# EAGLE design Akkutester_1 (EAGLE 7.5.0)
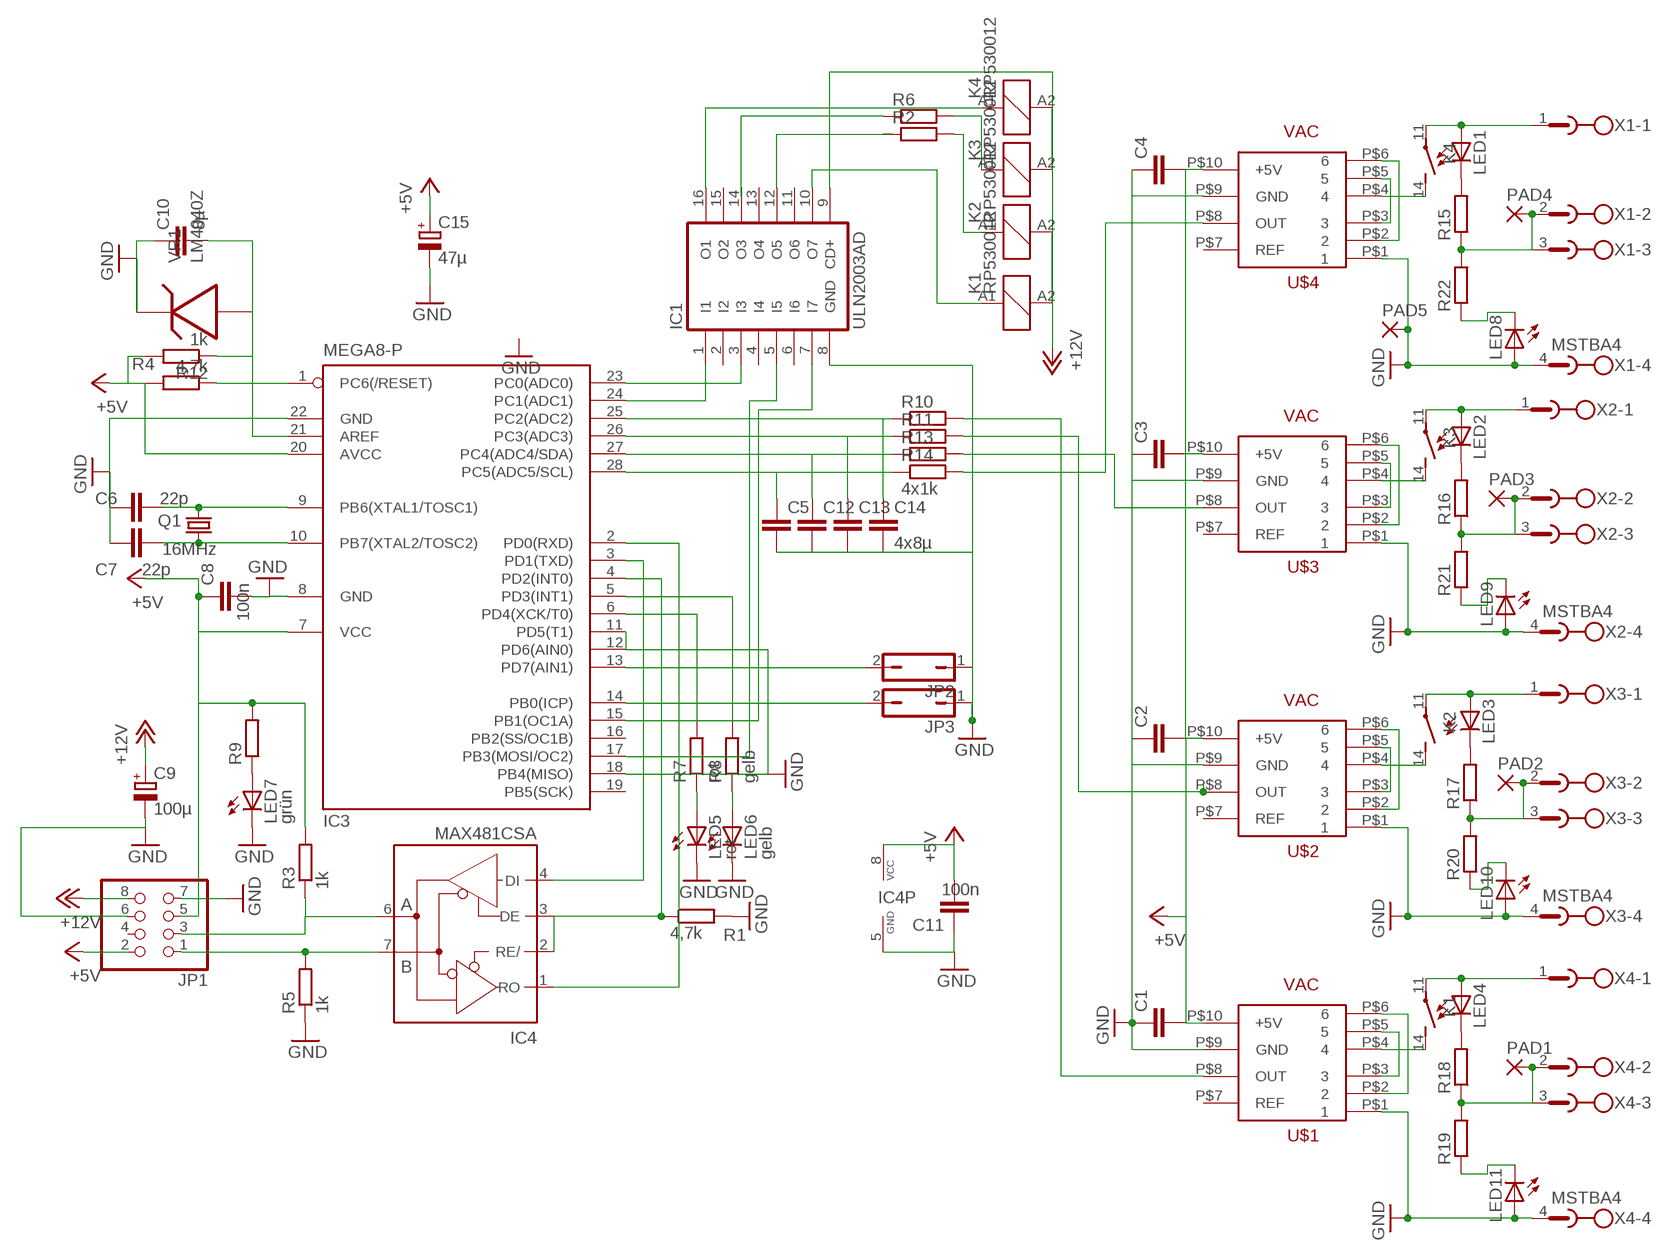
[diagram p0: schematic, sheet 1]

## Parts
C1  C-EUC0805  [C0805]
C2  C-EUC0805  [C0805]
C3  C-EUC0805  [C0805]
C4  C-EUC0805  [C0805]
C5  C-EUC0805  [C0805]
C6  22p  C-EUC0603  [C0603]
C7  22p  C-EUC0603  [C0603]
C8  100n  C-EUC0603  [C0603]
C9  100µ  CPOL-EUSMCD  [SMC_D]
C10  8µ  C-EUC0805  [C0805]
C11  100n  C-EU050-025X075  [C050-025X075]
C12  C-EUC0805  [C0805]
C13  C-EUC0805  [C0805]
C14  4x8µ  C-EUC0805  [C0805]
C15  47µ  CPOL-EUSMCD  [SMC_D]
IC1  ULN2003AD  [SO16]
IC3  MEGA8-P  [DIL28-3]
IC4  MAX481CSA  [SO08]
JP1  PINHD-2X4  [2X04]
JP2  JP1Q  [JP1]
JP3  JP1Q  [JP1]
K1  RP530012  [RP53]
K2  RP530012  [RP53]
K3  RP530012  [RP53]
K4  RP530012  [RP53]
LED1  LED3MM  [LED3MM]
LED2  LED3MM  [LED3MM]
LED3  LED3MM  [LED3MM]
LED4  LED3MM  [LED3MM]
LED5  rot  LEDCHIPLED_0603  [CHIPLED_0603]
LED6  gelb  LEDCHIPLED_0603  [CHIPLED_0603]
LED7  grün  LEDCHIPLED_0603  [CHIPLED_0603]
LED8  LED3MM  [LED3MM]
LED9  LED3MM  [LED3MM]
LED10  LED3MM  [LED3MM]
LED11  LED3MM  [LED3MM]
PAD1  1,6/0,9  [1,6/0,9]
PAD2  1,6/0,9  [1,6/0,9]
PAD3  1,6/0,9  [1,6/0,9]
PAD4  1,6/0,9  [1,6/0,9]
PAD5  1,6/0,9  [1,6/0,9]
Q1  16MHz  CRYSTALCTS406  [CTS406]
R1  4,7k  R-EU_R0603  [R0603]
R2  R-EU_R1206  [R1206]
R3  1k  R-EU_R0603  [R0603]
R4  4,7k  R-EU_R0603  [R0603]
R5  1k  R-EU_R1206  [R1206]
R6  R-EU_R1206  [R1206]
R7  rot  R-EU_R0603  [R0603]
R8  gelb  R-EU_R0603  [R0603]
R9  R-EU_R0603  [R0603]
R10  R-EU_R0603  [R0603]
R11  R-EU_R0603  [R0603]
R12  1k  R-EU_R0603  [R0603]
R13  R-EU_R0603  [R0603]
R14  4x1k  R-EU_R0603  [R0603]
R15  R-EU_R0603  [R0603]
R16  R-EU_R0603  [R0603]
R17  R-EU_R0603  [R0603]
R18  R-EU_R0603  [R0603]
R19  R-EU_R0603  [R0603]
R20  R-EU_R0603  [R0603]
R21  R-EU_R0603  [R0603]
R22  R-EU_R0603  [R0603]
U$1  VAC  [VAC]
U$2  VAC  [VAC]
U$3  VAC  [VAC]
U$4  VAC  [VAC]
VR1  LM4040Z  [TO92]
X1  MSTBA4  [MSTBA4]
X2  MSTBA4  [MSTBA4]
X3  MSTBA4  [MSTBA4]
X4  MSTBA4  [MSTBA4]

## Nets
+5V: C1.2 C2.2 C3.2 C4.2 C8.1 C11.2 C15.+ IC3.7(VCC) IC3.20(AVCC) IC4.8(VCC) JP1.2 JP1.5 R3.2 R4.2 R9.2 R12.2 U$1.P$10(+5V) U$2.P$10(+5V) U$3.P$10(+5V) U$4.P$10(+5V)
+12V: C9.+ IC1.9(CD+) JP1.8 K1.A2 K2.A2 K3.A2 K4.A2
GND: C1.1 C2.1 C3.1 C4.1 C5.2 C6.1 C7.1 C8.2 C9.- C10.1 C11.1 C12.2 C13.2 C14.2 C15.- IC1.8(GND) IC3.8(GND) IC3.11(PD5(T1)) IC3.12(PD6(AIN0)) IC3.18(PB4(MISO)) IC3.22(GND) IC4.5(GND) JP1.6 JP1.7 JP2.1 JP3.1 LED5.C LED6.C LED7.C LED8.A LED9.A LED10.A LED11.A PAD5.1(P) R1.2 R5.1 U$1.P$1 U$1.P$9(GND) U$2.P$1 U$2.P$9(GND) U$3.P$1 U$3.P$9(GND) U$4.P$1 U$4.P$9(GND) VR1.1 X1.4 X2.4 X3.4 X4.4
N$1: R14.2 U$4.P$8(OUT)
N$2: K1.14(2:S) U$1.P$4
N$3: IC1.1(I1) IC3.24(PC1(ADC1))
N$4: R11.2 U$2.P$8(OUT)
N$5: R10.2 U$1.P$8(OUT)
N$6: U$1.P$3 U$1.P$5
N$7: U$1.P$2 U$1.P$6
N$9: K2.14(2:S) U$2.P$4
N$10: U$2.P$3 U$2.P$5
N$11: U$2.P$2 U$2.P$6
N$13: K3.14(2:S) U$3.P$4
N$14: U$3.P$3 U$3.P$5
N$15: U$3.P$2 U$3.P$6
N$17: K4.11(2:P) LED1.A X1.1
N$18: PAD3.1(P) R16.1 R21.2 X2.2 X2.3
N$19: LED2.K(C) R16.2
N$20: K4.14(2:S) U$4.P$4
N$21: R13.2 U$3.P$8(OUT)
N$22: IC1.16(O1) K4.A1
N$23: K3.11(2:P) LED2.A X2.1
N$24: K2.11(2:P) LED3.A X3.1
N$25: K1.11(2:P) LED4.A X4.1
N$26: LED1.K(C) R15.2
N$28: IC4.6(A) JP1.3 R3.1
N$29: IC1.3(I3) IC3.23(PC0(ADC0))
N$30: C7.2 IC3.10(PB7(XTAL2/TOSC2)) Q1.1
N$31: U$4.P$3 U$4.P$5
N$32: U$4.P$2 U$4.P$6
N$33: PAD1.1(P) R18.1 R19.2 X4.2 X4.3
N$34: C6.2 IC3.9(PB6(XTAL1/TOSC1)) Q1.3
N$35: IC3.4(PD2(INT0)) IC4.2(RE/) IC4.3(DE) R1.1
N$36: IC3.1(PC6(/RESET)) R4.1
N$37: IC3.2(PD0(RXD)) IC4.1(RO)
N$38: IC3.3(PD1(TXD)) IC4.4(DI)
N$39: IC3.14(PB0(ICP)) JP3.2
N$40: IC3.13(PD7(AIN1)) JP2.2
N$41: IC3.6(PD4(XCK/T0)) R7.2
N$42: IC3.5(PD3(INT1)) R8.2
N$43: LED5.A R7.1
N$44: LED6.A R8.1
N$45: K2.A1 R2.2
N$46: IC1.5(I5) IC3.17(PB3(MOSI/OC2))
N$47: IC1.7(I7) IC3.15(PB1(OC1A))
N$48: LED7.A R9.1
N$49: IC1.14(O3) R6.1
N$50: IC1.10(O7) K1.A1
N$51: C10.2 IC3.21(AREF) R12.1 VR1.2
N$52: IC1.12(O5) R2.1
N$53: C14.1 IC3.25(PC2(ADC2)) R10.1
N$54: K3.A1 R6.2
N$55: C13.1 IC3.26(PC3(ADC3)) R11.1
N$56: C12.1 IC3.27(PC4(ADC4/SDA)) R13.1
N$57: C5.1 IC3.28(PC5(ADC5/SCL)) R14.1
N$58: IC4.7(B) JP1.1 R5.2
N$59: PAD4.1(P) R15.1 R22.2 X1.2 X1.3
N$60: PAD2.1(P) R17.1 R20.2 X3.2 X3.3
N$61: LED3.K(C) R17.2
N$62: LED4.K(C) R18.2
N$63: LED11.K(C) R19.1
N$64: LED10.K(C) R20.1
N$65: LED9.K(C) R21.1
N$66: LED8.K(C) R22.1
Unconnected: IC1.2(I2) IC1.4(I4) IC1.6(I6) IC1.11(O6) IC1.13(O4) IC1.15(O2) IC3.16(PB2(SS/OC1B)) IC3.19(PB5(SCK)) JP1.4 U$1.P$7(REF) U$2.P$7(REF) U$3.P$7(REF) U$4.P$7(REF)

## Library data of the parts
C1-C8 C10-C14 = rcl:C-EU: CAPACITOR, European symbol
C9 C15 = rcl:CPOL-EU: POLARIZED CAPACITOR, European symbol
IC1 = uln-udn:ULN2003A: DRIVER ARRAY
IC3 = atmel:MEGA8-P: MICROCONTROLLER 8 Kbytes FLASH, 1 kbytes SRAM, 512 bytes EEPROM, USART, 4-channel 10 bit ADC, 2-channel 8 bit ADC Pin compatible with Atmega48, ATMega88, ATMega168 Source: avr.lbr
IC4 = maxim:MAX481CSA: RS485 TRANSEIVER
JP1 = pinhead:PINHD-2X4: PIN HEADER
JP2 JP3 = jumper:JP1Q: JUMPER
K1-K4 = relay:RP53*: Power PCB Relay RP I SCHRACK 1 pole 8 A Vertical version Source: http://www.schrack.com/.. 5845.pdf
LED1-LED11 = led:LED: LED
PAD1-PAD5 = wirepad:1,6/0,9: THROUGH-HOLE PAD
Q1 = crystal:CRYSTAL: CRYSTAL
R1-R22 = rcl:R-EU_: RESISTOR, European symbol
U$1-U$4 = VAC:VAC
VR1 = synthdiy:LM4040: Shunt VOLTAGE REG.
X1-X4 = con-phoenix-508:MSTBA4: PHOENIX

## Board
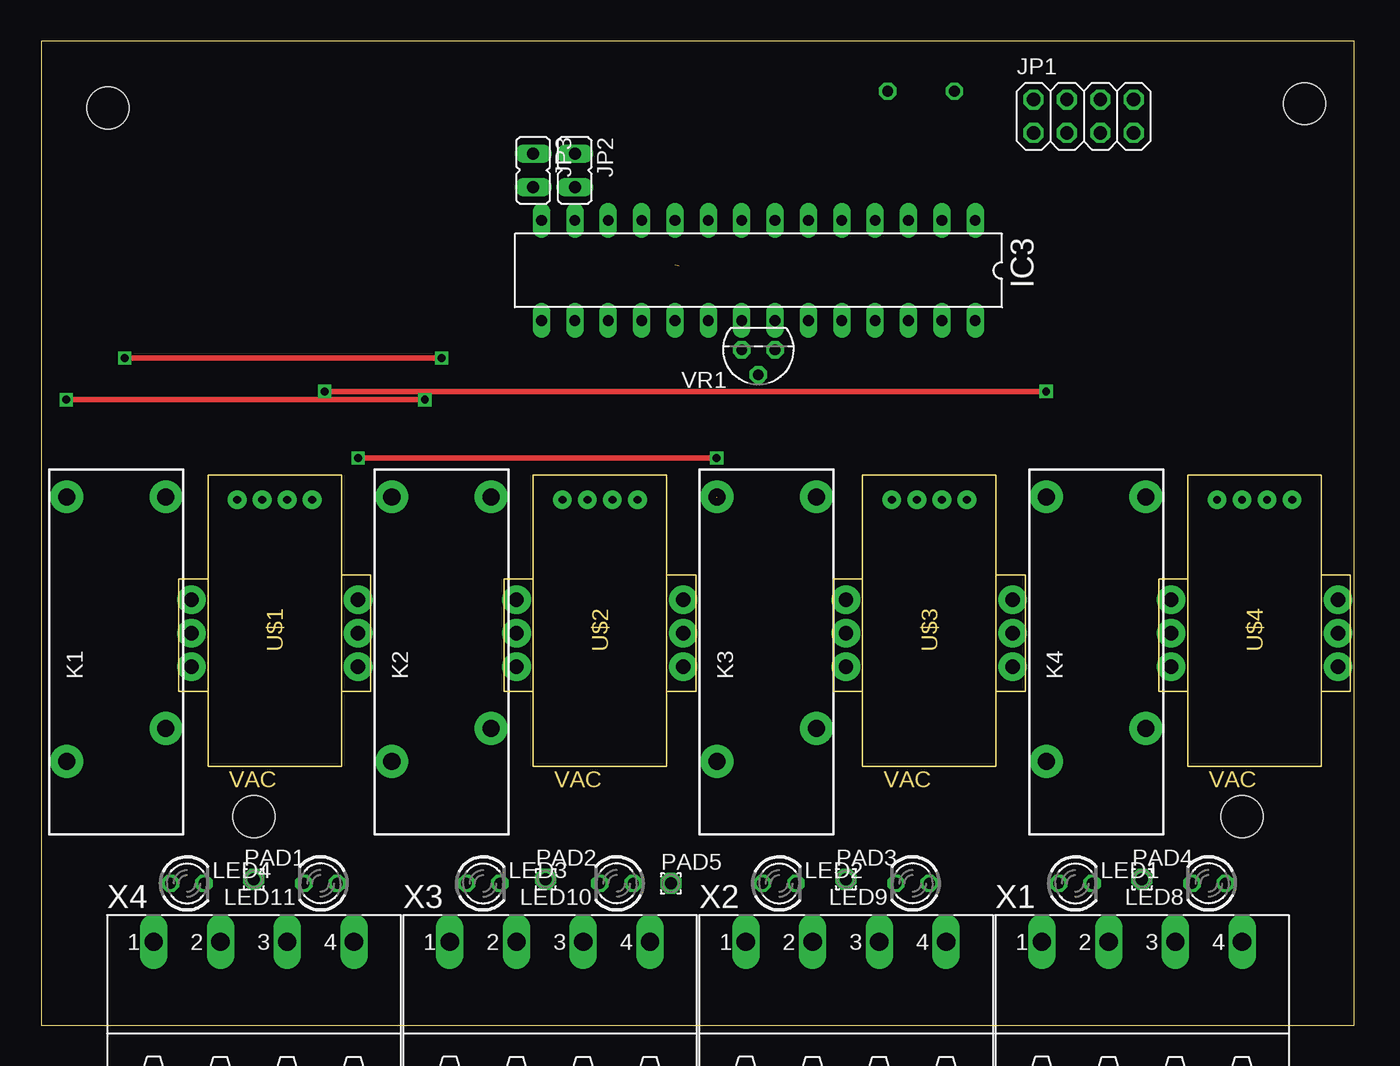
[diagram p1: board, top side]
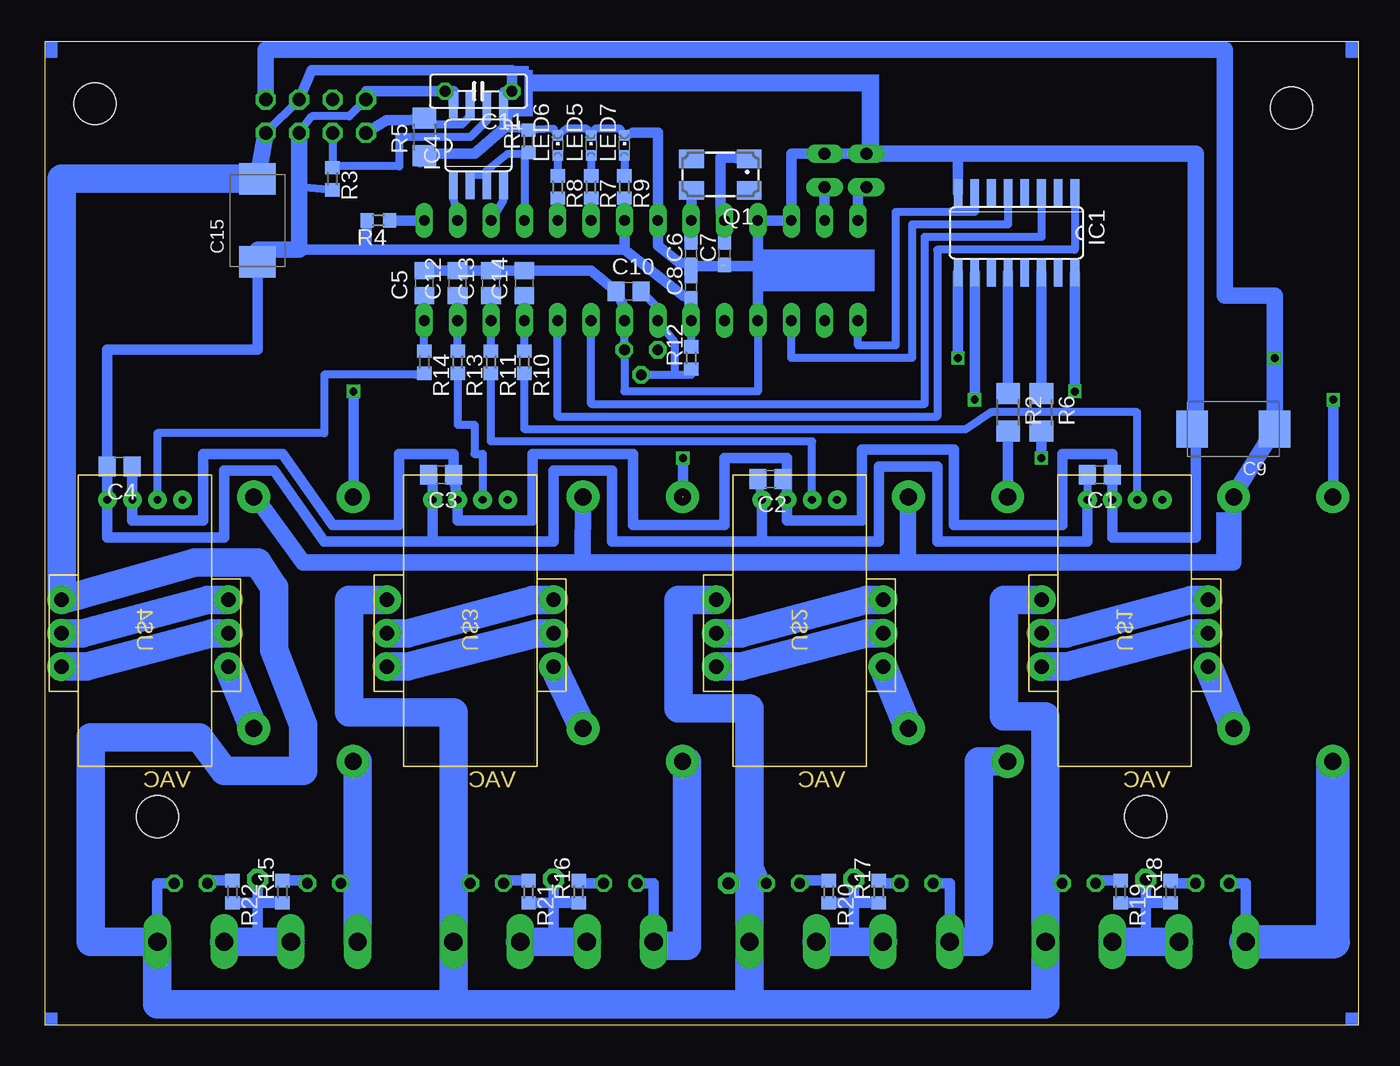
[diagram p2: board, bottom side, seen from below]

Size 100 x 74.92 mm. Coordinates in mm from the lower left corner, seen from the top.
Outline: 0,0 100,0 100,74.92 0,74.92 0,0
Copper layers (1*16): Top 0.035mm / dielectric 1.5mm / Bottom 0.035mm
Design rules "default": minimum track width 10mil, minimum drill 24mil, track to track 8mil, track to pad 8mil, pad to pad 8mil, via to via 8mil, smd to smd 8mil, copper to edge 40mil, drill to drill 8mil, minimum pad ring 10mil, minimum via ring 8mil, stop-mask expansion 4mil, vias tented up to drill 0mil, thermal gap 10mil
Holes 3.2 mm at 16.19,15.88 91.44,15.88 5.08,69.85 96.2,70.17

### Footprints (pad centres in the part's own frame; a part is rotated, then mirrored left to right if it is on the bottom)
C0805 = smd 1.3 x 1.5: 1 -0.95,0; 2 0.95,0
C0603 = smd 1.1 x 1: 1 -0.85,0; 2 0.85,0
SMC_D = smd 2.4 x 2.8: + -3.15,0; - 3.15,0
C050-025X075 = drill 0.813 octagon: 1 -2.54,0; 2 2.54,0
SO16 = smd 0.66 x 2.032: 1 -4.445,-3.073; 2 -3.175,-3.073; 3 -1.905,-3.073; 4 -0.635,-3.073; 5 0.635,-3.073; 6 1.905,-3.073; 7 3.175,-3.073; 8 4.445,-3.073; 9 4.445,3.073; 10 3.175,3.073; 11 1.905,3.073; 12 0.635,3.073; 13 -0.635,3.073; 14 -1.905,3.073; 15 -3.175,3.073; 16 -4.445,3.073
DIL28-3 = drill 0.813 long: 1 -16.51,-3.81; 2 -13.97,-3.81; 3 -11.43,-3.81; 4 -8.89,-3.81; 5 -6.35,-3.81; 6 -3.81,-3.81; 7 -1.27,-3.81; 8 1.27,-3.81; 9 3.81,-3.81; 10 6.35,-3.81; 11 8.89,-3.81; 12 11.43,-3.81; 13 13.97,-3.81; 14 16.51,-3.81; 15 16.51,3.81; 16 13.97,3.81; 17 11.43,3.81; 18 8.89,3.81; 19 6.35,3.81; 20 3.81,3.81; 21 1.27,3.81; 22 -1.27,3.81; 23 -3.81,3.81; 24 -6.35,3.81; 25 -8.89,3.81; 26 -11.43,3.81; 27 -13.97,3.81; 28 -16.51,3.81
SO08 = smd 0.66 x 2.032: 1 -1.905,-3.073; 2 -0.635,-3.073; 3 0.635,-3.073; 4 1.905,-3.073; 5 1.905,3.073; 6 0.635,3.073; 7 -0.635,3.073; 8 -1.905,3.073
2X04 = drill 1.016 octagon: 1 -3.81,-1.27; 2 -3.81,1.27; 3 -1.27,-1.27; 4 -1.27,1.27; 5 1.27,-1.27; 6 1.27,1.27; 7 3.81,-1.27; 8 3.81,1.27
JP1 = drill 0.914 long: 1 0,-1.27; 2 0,1.27
RP53 = drill 1.3 pad 2.5: 11 -8.82,3.78; 14 -6.3,-3.78; A1 11.34,3.78; A2 11.34,-3.78
LED3MM = drill 0.813 octagon: A -1.27,0; K 1.27,0
CHIPLED_0603 = smd 0.8 x 0.8: A 0,-0.75; C 0,0.75
1,6/0,9 = drill 0.914 pad 1.6 octagon: 1 0,0
CTS406 = smd 1.9 x 1.4: 1 -2.2,-1.2; 2 2.2,-1.2; 3 2.2,1.2; 4 -2.2,1.2
R0603 = smd 1 x 1.1: 1 -0.85,0; 2 0.85,0
R1206 = smd 1.6 x 1.803: 1 -1.422,0; 2 1.422,0
VAC = drill 1.1 pad 2.184: P$1 1.27,6.35; P$2 3.81,6.35; P$3 6.35,6.35; P$4 6.35,-6.35; P$5 3.81,-6.35; P$6 1.27,-6.35 | drill 0.6 pad 1.422: P$7 -6.35,-2.857; P$8 -6.35,-0.953; P$9 -6.35,0.953; P$10 -6.35,2.857
TO92 = drill 0.813 octagon: 1 -1.27,0; 2 0,1.905; 3 1.27,0
MSTBA4 = drill 1.397 long: 1 -7.62,5.08; 2 -2.54,5.08; 3 2.54,5.08; 4 7.62,5.08

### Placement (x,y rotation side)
C1  19.68,41.91 180 bottom
C2  44.77,41.59 180 bottom
C3  69.85,41.91 180 bottom
C4  94.3,42.55 180 bottom
C5  71.12,56.52 90 bottom
C6  50.8,58.74 90 bottom
C7  48.26,58.74 90 bottom
C8  50.8,56.2 90 bottom
C9  9.53,45.4 180 bottom
C10  55.56,55.88 0 bottom
C11  66.99,71.12 180 bottom
C12  68.58,56.52 90 bottom
C13  66.04,56.52 90 bottom
C14  63.5,56.52 90 bottom
C15  83.82,61.28 90 bottom
IC1  26.04,60.33 180 bottom
IC3  54.61,57.47 180 top
IC4  66.99,66.99 0 bottom
JP1  79.38,69.22 0 top
JP2  40.64,65.09 180 top
JP3  37.47,65.09 180 top
K1  5.71,28.89 90 top
K2  30.48,28.89 90 top
K3  55.24,28.89 90 top
K4  80.33,28.89 90 top
LED1  78.74,10.79 0 top
LED2  56.2,10.79 0 top
LED3  33.66,10.79 0 top
LED4  11.11,10.79 0 top
LED5  58.42,66.99 0 bottom
LED6  60.96,66.99 0 bottom
LED7  55.88,66.99 0 bottom
LED8  88.9,10.79 180 top
LED9  66.36,10.79 180 top
LED10  43.81,10.79 180 top
LED11  21.27,10.79 180 top
PAD1  16.19,11.11 0 top
PAD2  38.42,11.11 0 top
PAD3  61.28,11.11 0 top
PAD4  83.82,11.11 0 top
PAD5  47.94,10.79 0 top
Q1  48.58,64.77 180 bottom
R1  63.18,67.31 90 bottom
R2  26.67,46.67 270 bottom
R3  78.11,64.45 270 bottom
R4  74.61,61.28 180 bottom
R5  71.12,67.63 90 bottom
R6  24.13,46.67 270 bottom
R7  58.42,63.82 270 bottom
R8  60.96,63.82 270 bottom
R9  55.88,63.82 270 bottom
R10  63.5,50.48 270 bottom
R11  66.04,50.48 270 bottom
R12  50.8,50.8 90 bottom
R13  68.58,50.48 270 bottom
R14  71.12,50.48 270 bottom
R15  81.92,10.16 90 bottom
R16  59.37,10.16 90 bottom
R17  36.51,10.16 90 bottom
R18  14.29,10.16 90 bottom
R19  18.1,10.16 270 bottom
R20  40.32,10.16 270 bottom
R21  63.18,10.16 270 bottom
R22  85.72,10.16 270 bottom
U$1  17.78,33.66 270 top
U$2  42.55,33.66 270 top
U$3  67.63,33.66 270 top
U$4  92.39,33.66 270 top
VR1  54.61,51.44 180 top
X1  83.82,1.27 0 top
X2  61.28,1.27 0 top
X3  38.73,1.27 0 top
X4  16.19,1.27 0 top

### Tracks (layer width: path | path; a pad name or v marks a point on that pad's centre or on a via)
+5V
  Bottom 0.61: IC3.20 R12.2 | JP1.2 76.83,69.22 79.69,69.22 JP1.5 | C15.+ 83.82,59.05 | R3.2 80.64,63.82 | C1.2 U$1.P$10 | U$2.P$10 C2.2 | U$4.P$10 C4.2
  Bottom 0.813: R9.2 IC3.7 55.88,59.05 | 75.56,59.05 55.88,59.05 | R4.2 75.56,59.05 | IC3.20 C8.1 51.44,55.56 55.88,59.05 | IC4.8 68.9,71.12 C11.2 75.56,71.12 JP1.2 | 75.56,59.05 80.64,59.05 | C15.+ 83.82,51.44 95.25,51.44 U$4.P$10 | C3.2 70.48,41.91 U$3.P$10 70.48,36.83 | U$1.P$10 20.64,36.83 32.07,36.83 32.07,42.55 36.51,42.55 36.51,36.83 45.4,36.83 | U$2.P$10 45.4,36.83 | 45.4,36.83 56.83,36.83 56.83,42.23 61.28,42.23 61.28,36.83 70.48,36.83 | C4.2 95.25,37.15 86.36,37.15 86.36,42.23 82.55,42.23 78.74,36.83 70.48,36.83
  Bottom 1.27: JP1.5 80.64,63.82 80.64,59.05 83.82,59.05
+12V  (via drill 0.6)
  Top 0.406: v30.48,50.8 v6.35,50.8
  Bottom 0.813: IC1.9 v30.48,50.8 | v6.35,50.8 C9.+
  Bottom 1.27: 34.29,35.24 9.53,35.24 9.53,39.05 K1.A2 9.53,40.32 C9.+ 6.35,55.56 10.16,55.56 10.16,74.3 83.19,74.3 JP1.8 | 59.05,35.24 80.33,35.24 83.82,40.01 K4.A2 | K3.A2 59.05,35.24 | K2.A2 34.29,39.05 34.29,35.24 | 34.29,35.24 59.05,35.24
GND  (1 unrouted)
  Bottom 0.61: IC3.18 45.72,48.26 55.88,48.26 VR1.1 IC3.22 | LED7.C 56.2,68.26 58.1,68.26 LED5.C 58.74,68.26 60.33,68.26 LED6.C 61.28,68.26 R1.2 63.82,68.26 65.09,68.26 IC4.5 65.09,71.12 C11.1 | C8.2 C6.1 | JP1.6 JP1.7 | C2.1 43.5,41.59
  Bottom 0.813: IC1.8 30.48,66.36 JP3.1 JP2.1 43.18,66.36 IC3.12 IC3.11 45.72,57.78 | 45.72,57.78 IC3.18 | 48.58,57.78 50.16,57.78 C6.1 51.75,58.1 53.34,59.37 IC3.8 53.34,67.94 55.24,67.94 LED7.C | C7.1 47.94,57.78 45.72,57.78 | C5.2 C12.2 C13.2 C14.2 62.87,57.47 58.42,57.47 C10.1 55.88,54.61 IC3.22 | 65.09,68.26 67.31,66.36 71.12,66.36 R5.1 71.44,65.72 | JP1.6 79.69,72.71 64.45,72.71 C11.1 | 12.38,45.72 C9.- 12.38,44.13 12.38,37.15 18.73,37.15 C1.1 18.73,42.86 | U$1.P$9 18.73,42.86 | 18.73,42.86 18.73,43.5 22.54,43.5 22.54,38.1 30.8,38.1 30.8,43.81 37.78,43.81 37.78,38.42 43.5,38.42 U$2.P$9 43.5,41.59 43.5,43.18 48.26,43.18 48.26,38.1 55.24,38.1 55.24,43.5 62.87,43.5 62.87,38.42 68.58,38.42 U$3.P$9 C3.1 68.9,43.5 73.03,43.5 73.03,38.1 78.11,38.1 81.92,43.5 87.95,43.5 87.95,38.42 93.34,38.42 C4.1 U$4.P$9 | LED9.A 68.9,11.11 | LED10.A 46.35,13.65 | X4.4 23.81,6.99 23.81,10.79 LED11.A | X1.4 91.44,10.79 LED8.A | PAD5.1 46.35,10.79
  Bottom 1.27: JP1.7 83.82,64.45 83.19,65.09 C15.- | 12.38,45.72 12.38,66.36 JP3.1
  Bottom 2.184: U$3.P$1 76.83,32.38 76.83,23.81 68.9,23.81 68.9,11.11 X2.4 68.9,1.59 | U$2.P$1 51.75,32.38 51.75,24.13 46.35,24.13 46.35,13.65 46.35,10.79 X3.4 46.35,1.59 | U$1.P$1 26.99,32.38 26.99,23.5 23.81,23.5 23.81,6.99 | U$4.P$1 97.47,32.7 88.58,35.24 83.82,35.24 82.55,33.34 82.55,28.57 80.33,22.86 80.33,19.37 86.36,19.37 88.27,21.91 96.52,21.91 96.52,6.35 X1.4 91.44,1.59 68.9,1.59 | 98.74,35.24 U$4.P$1 | U$4.P$1 98.74,64.45 83.82,64.45 | 68.9,1.59 46.35,1.59 | 46.35,1.59 23.81,1.59 X4.4
N$1
  Bottom 0.61: R14.2 71.75,49.53 78.74,49.53 78.74,45.09 91.44,45.09 U$4.P$8
N$2
  Bottom 2.184: K1.14 U$1.P$4
N$3
  Bottom 0.61: IC1.1 21.59,59.05 32.07,59.05 32.07,46.35 60.96,46.35 IC3.24
N$4
  Bottom 0.61: U$2.P$8 41.59,44.45 66.04,44.45 R11.2
N$5
  Bottom 0.61: R10.2 63.5,45.4 29.84,45.4 27.94,46.67 16.83,46.67 U$1.P$8
N$6
  Bottom 2.184: U$1.P$5 12.7,29.84 22.23,27.3 U$1.P$3
N$7
  Bottom 2.184: U$1.P$6 12.7,32.38 22.23,29.84 U$1.P$2
N$9
  Bottom 2.184: K2.14 U$2.P$4
N$10
  Bottom 2.184: U$2.P$5 37.47,29.84 46.99,27.3 U$2.P$3
N$11
  Bottom 2.184: U$2.P$6 37.47,32.38 46.99,29.84 U$2.P$2
N$13
  Bottom 2.184: K3.14 U$3.P$4
N$14
  Bottom 2.184: U$3.P$5 62.55,29.84 72.39,27.3 U$3.P$3
N$15
  Bottom 2.184: U$3.P$6 62.87,32.38 72.39,29.84 U$3.P$2
N$17
  Bottom 0.813: LED1.A 76.2,10.79 X1.1
  Bottom 2.184: K4.11 76.2,20.07 X1.1
N$18
  Bottom 0.813: R21.2 61.28,9.31 | 61.28,9.31 R16.1 | X2.3 61.28,6.03 61.28,8.89 61.28,9.31 | PAD3.1 61.28,9.31
  Bottom 2.184: X2.2 X2.3
N$19
  Bottom 0.813: LED2.K 59.37,10.79 R16.2
N$20
  Bottom 2.184: K4.14 U$4.P$4
N$21
  Bottom 0.61: R13.2 68.58,45.72 67.31,45.72 67.31,43.5 66.67,43.5 U$3.P$8
N$22  (via drill 0.6)
  Top 0.406: v76.52,48.26 v21.59,48.26
  Bottom 0.813: K4.A1 76.52,40.23 v76.52,48.26 | v21.59,48.26 IC1.16
N$23
  Bottom 0.813: X2.1 53.66,10.79 LED2.A
  Bottom 2.184: K3.11 51.12,20.07 51.12,6.03 53.66,6.03 X2.1
N$24
  Bottom 0.813: X3.1 31.11,10.79 LED3.A
  Bottom 2.184: K2.11 28.89,20.07 28.89,6.35 X3.1
N$25
  Bottom 0.813: X4.1 8.57,10.79 LED4.A
  Bottom 2.54: X4.1 1.94,6.35 | 1.91,6.35 1.94,6.35 | 1.94,6.35 K1.11
N$26
  Bottom 0.813: R15.2 80.01,11.01 LED1.K
N$28
  Bottom 0.61: IC4.6 66.36,68.9 67.63,67.63 73.03,67.63 73.03,65.41 77.79,65.41 R3.1 JP1.3
N$29
  Bottom 0.61: IC1.3 24.13,60.01 33.02,60.01 33.02,47.31 58.42,47.31 IC3.23
N$30
  Bottom 0.813: C7.2 IC3.10 48.58,61.91 48.58,66.04 Q1.1
N$31
  Bottom 2.184: U$4.P$5 87.31,29.84 96.84,27.3 U$4.P$3
N$32
  Bottom 2.184: U$4.P$6 87.63,32.38 97.16,29.84 U$4.P$2
N$33
  Bottom 0.813: R18.1 16.19,9.31 | 16.19,9.31 R19.2 | X4.3 16.19,6.03 16.19,8.26 16.19,9.31 | PAD1.1 16.19,9.31
  Bottom 2.184: X4.2 X4.3
N$34
  Bottom 0.813: Q1.3 IC3.9 C6.2
N$35
  Bottom 0.61: IC4.2 67.63,64.77 66.36,64.77 | IC4.3 66.36,64.77 | IC3.4 63.5,66.36 R1.1 63.82,66.36 64.77,66.36 66.36,65.09 66.36,64.77
N$36
  Bottom 0.813: IC3.1 R4.1
N$37
  Bottom 0.61: IC4.1 68.9,62.87 IC3.2
N$38
  Bottom 0.61: IC4.4 65.09,62.87 IC3.3
N$39
  Bottom 0.813: JP3.2 38.1,63.82 IC3.14
N$40
  Bottom 0.813: JP2.2 IC3.13
N$41
  Bottom 0.813: IC3.6 R7.2
N$42
  Bottom 0.813: IC3.5 R8.2
N$43
  Bottom 0.61: LED5.A R7.1
N$44
  Bottom 0.61: LED6.A R8.1
N$45
  Bottom 0.813: K2.A1 26.67,40.23 R2.2
N$46
  Bottom 0.61: IC3.17 43.18,50.8 33.97,50.8 33.97,60.96 26.67,60.96 IC1.5
N$47
  Bottom 0.61: IC1.7 29.21,61.91 35.24,61.91 35.24,51.75 38.1,51.75 IC3.15
N$48
  Bottom 0.61: LED7.A R9.1
N$49
  Bottom 0.813: IC1.14 R6.1
N$50  (via drill 0.6)
  Top 0.406: v1.91,47.62 v29.21,47.62
  Bottom 0.813: K1.A1 1.91,40.23 v1.91,47.62 | v29.21,47.62 IC1.10
N$51
  Bottom 0.61: VR1.2 52.07,49.53 | 52.07,49.53 50.8,49.53 R12.1 | 52.07,49.53 52.07,52.07 IC3.21 53.34,54.61 C10.2
N$52
  Bottom 0.813: R2.1 IC1.12
N$53
  Bottom 0.61: R10.1 IC3.25 C14.1
N$54  (via drill 0.6)  (1 unrouted)
  Top 0.406: v51.44,43.18 v24.13,43.18
  Bottom 0.813: 51.44,40.23 v51.44,43.18 | v24.13,43.18 R6.2
N$55
  Bottom 0.61: R11.1 IC3.26 C13.1
N$56
  Bottom 0.61: R13.1 IC3.27 C12.1
N$57
  Bottom 0.61: R14.1 IC3.28 C5.1
N$58
  Bottom 0.61: 71.12,69.53 R5.2 | 71.75,68.58 R5.2 | IC4.7 67.63,69.22 68.26,68.58 70.17,68.58 R5.2
  Bottom 0.813: JP1.1 73.98,68.9 72.39,68.9 R5.2
N$59
  Bottom 0.813: R22.2 83.82,9.31 | 83.82,9.31 R15.1 | 83.82,6.35 83.82,9.31 | PAD4.1 83.82,9.31
  Bottom 2.184: X1.2 83.82,6.35 X1.3
N$60
  Bottom 0.813: R17.1 38.42,9.31 | 38.42,9.31 R20.2 | 38.42,6.35 38.42,9.31 | PAD2.1 38.42,9.31
  Bottom 2.184: X3.2 38.42,6.35 X3.3
N$61
  Bottom 0.813: LED3.K 35.88,10.79 R17.2
N$62
  Bottom 0.813: LED4.K 14.29,10.79 R18.2
N$63
  Bottom 0.813: R19.1 20,11.01 LED11.K
N$64
  Bottom 0.813: R20.1 42.55,11.01 LED10.K
N$65
  Bottom 0.813: R21.1 65.09,11.01 LED9.K
N$66
  Bottom 0.813: R22.1 87.63,11.01 LED8.K
(copper drawn outside any net)
  shapes: Bottom area x18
